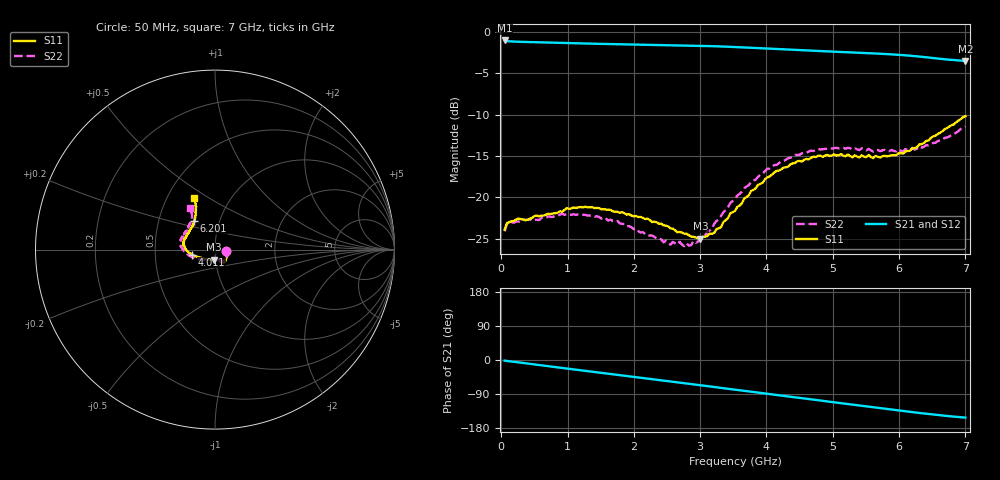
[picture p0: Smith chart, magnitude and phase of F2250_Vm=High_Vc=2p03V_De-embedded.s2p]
! Integrated Device Technology
! Corporate Headquarters
! 6024 Silver Creek Valley Road
! San Jose, CA 95138  USA
! Phone:  1-408-284-8200
! Toll Free:  1-800-223-1366
! Webpage:  http://www.idt.com/
! Timing and RF Division
! 515 Groton Road, Suite 102
! Westford, MA 01886-6024
! Device:  F2250
! Description: Voltage Variable RF Attenuator
! Frequency:  50.0 -  6000.00 MHz
! Package:  3x3 mm Thin QFN Plastic Package: 16 pin
! Ports:  2 RF, 3 DC
!  Pin  1  = GND
!  Pin  2  = NC
!  Pin  3  = RF1  = Port 1
!  Pin  4  = NC
!  Pin  5  = GND
!  Pin  6  = GND
!  Pin  7  = GND
!  Pin  8  = GND
!  Pin  9  = NC
!  Pin 10  = RF2  = Port 2
!  Pin 11  = NC
!  Pin 12  = GND
!  Pin 13  = GND
!  Pin 14  = VCNTRL
!  Pin 15  = VDD
!  Pin 16  = VMODE
! Vcntrl:  2.030 Volts
! Vmode:  +3.300 Volts
! Vdd:  +3.30  Volts
! Current:  1.319 mA
! Data:  The device was measured on a the F2250 evaluation board which has
!  individual transmission lines to the RF pins.  Data was collected
!  using a calibrated network analyzer.  The evaluation board was
!  de-embedded using a TRL calibration technique.
!  The reference plane is the edge of the package pin.
! Misc:  SN 10
!  Action Tracker AT0258
! Date Measured:  2014-11-26
! Date:  2015-10-15  MJV
! Note:
!  Integrated Device Technology supplies this data as a sample of measured
!  data at the package pin for this product.  Your particular data for this
!  product may vary.
!  Data was taken at 25 degrees C.
!  Integrated Device Technology reserves the right to change this data at anytime.
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# GHz S dB R 50
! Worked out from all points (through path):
!   201 points, 50 MHz to 7 GHz, reference 50 ohm
!   highest |S21| = -1.01 dB at 50 MHz (marker M1); lowest = -3.5 dB at 7 GHz (marker M2)
!   group delay of S21, straight-line fit = 61.1 ps
!   lowest |S11| = -25.0 dB at 3.004 GHz (marker M3), VSWR 1.12, Z = 49.3 - j5.55 ohm
!   |S11| at or under -10 dB: start of sweep to end of sweep
!   |S22| runs from -25.9 to -11.4 dB; largest |S21 - S12| = 0.0019
!   S11 on the Smith chart (normalised r, x): 50 MHz: 1.13, -0.02; 4.011 GHz: 0.77, -0.04; 6.201 GHz: 0.75, +0.25; 7 GHz: 0.68, +0.43
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0.05  -23.89 -8.8  -1.01 -1.8  -1.00 -1.8  -24.11 -9.5
0.08475  -23.12 -8.0  -1.08 -2.5  -1.08 -2.5  -23.22 -8.5
0.1195  -23.00 -8.7  -1.11 -3.3  -1.11 -3.2  -23.03 -8.0
0.91875  -21.73 -44.6  -1.30 -21.0  -1.30 -21.1  -21.99 -47.8
1.2315  -21.20 -52.4  -1.37 -27.9  -1.37 -27.9  -22.10 -58.1
1.75275  -21.75 -59.3  -1.46 -39.1  -1.46 -39.1  -22.85 -66.0
2.37825  -23.18 -59.9  -1.55 -52.7  -1.55 -52.8  -24.91 -69.5
2.552  -23.76 -64.2  -1.57 -56.6  -1.57 -56.6  -25.73 -76.0
2.691  -24.18 -70.9  -1.60 -59.7  -1.60 -59.7  -25.37 -83.0
2.7605  -24.39 -72.6  -1.61 -61.2  -1.61 -61.3  -25.90 -87.2
3.00375  -24.99 -94.4  -1.66 -66.7  -1.66 -66.7  -24.87 -108.9
3.21225  -24.29 -116.3  -1.70 -71.4  -1.70 -71.4  -23.19 -127.3
3.525  -21.64 -144.0  -1.80 -78.5  -1.80 -78.5  -20.18 -146.0
3.76825  -19.22 -158.5  -1.89 -84.0  -1.89 -84.0  -18.14 -157.4
4.0115  -17.57 -167.9  -1.99 -89.4  -1.99 -89.4  -16.54 -167.1
4.4285  -15.84 -180.0  -2.15 -98.6  -2.16 -98.6  -14.87 -179.9
4.7065  -15.07 172.7  -2.25 -104.8  -2.25 -104.8  -14.38 174.2
5.054  -14.92 164.4  -2.38 -112.4  -2.37 -112.5  -14.00 166.9
5.85325  -14.99 138.1  -2.68 -129.9  -2.68 -130.0  -14.40 147.9
6.20075  -14.03 126.0  -2.88 -137.6  -2.88 -137.7  -14.01 138.8
6.54825  -12.55 117.5  -3.15 -144.7  -3.16 -144.8  -13.39 127.4
7  -10.18 112.3  -3.48 -152.0  -3.49 -152.1  -11.41 121.0
